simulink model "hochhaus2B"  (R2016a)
settings: Solver=ode45  StartTime=0.0  StopTime=5  MaxStep=3e-3  RelTol=1e-3
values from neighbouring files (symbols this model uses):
  m = 1.0    (= 1)    [init_pendelStange.m]
undefined symbols (not defined in the file or in its folder): v0, x0

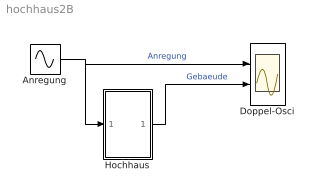
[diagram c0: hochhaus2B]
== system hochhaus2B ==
  Anregung : Sin  Amplitude=1e3  Frequency=12  SampleTime=0
  Doppel-Osci : Scope  NumInputPorts=2
  Hochhaus : Subsystem
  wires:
  Anregung/1 -> Doppel-Osci/1, Hochhaus/1(F)  "Anregung"
  Hochhaus/1(x) -> Doppel-Osci/2  "Gebaeude"

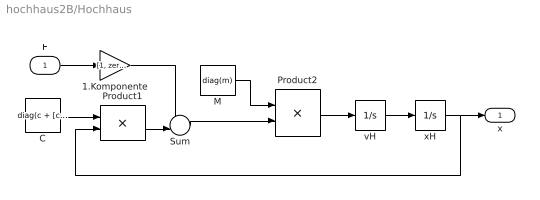
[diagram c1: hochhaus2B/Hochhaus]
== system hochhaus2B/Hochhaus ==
  F : Inport
  1.Komponente : Gain  Gain=[1, zeros(1,length(m)-1)]
  C : Constant  Value=diag(c + [c(2:end),0]) - diag(c(2:end),1) - diag(c(2:end),-1)  VectorParams1D=off
  M : Constant  Value=diag(m)  VectorParams1D=off
  Product1 : Product  Multiplication=Matrix(*)
  Product2 : Product  Inputs=/*  Multiplication=Matrix(*)
  Sum : Sum  Inputs=+-|
  vH : Integrator  InitialCondition=v0
  xH : Integrator  InitialCondition=x0
  x : Outport
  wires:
  vH/1 -> xH/1
  xH/1 -> Product1/2, x/1
  Product1/1 -> Sum/2
  C/1 -> Product1/1
  Sum/1 -> Product2/2
  Product2/1 -> vH/1
  M/1 -> Product2/1
  F/1 -> 1.Komponente/1
  1.Komponente/1 -> Sum/1
